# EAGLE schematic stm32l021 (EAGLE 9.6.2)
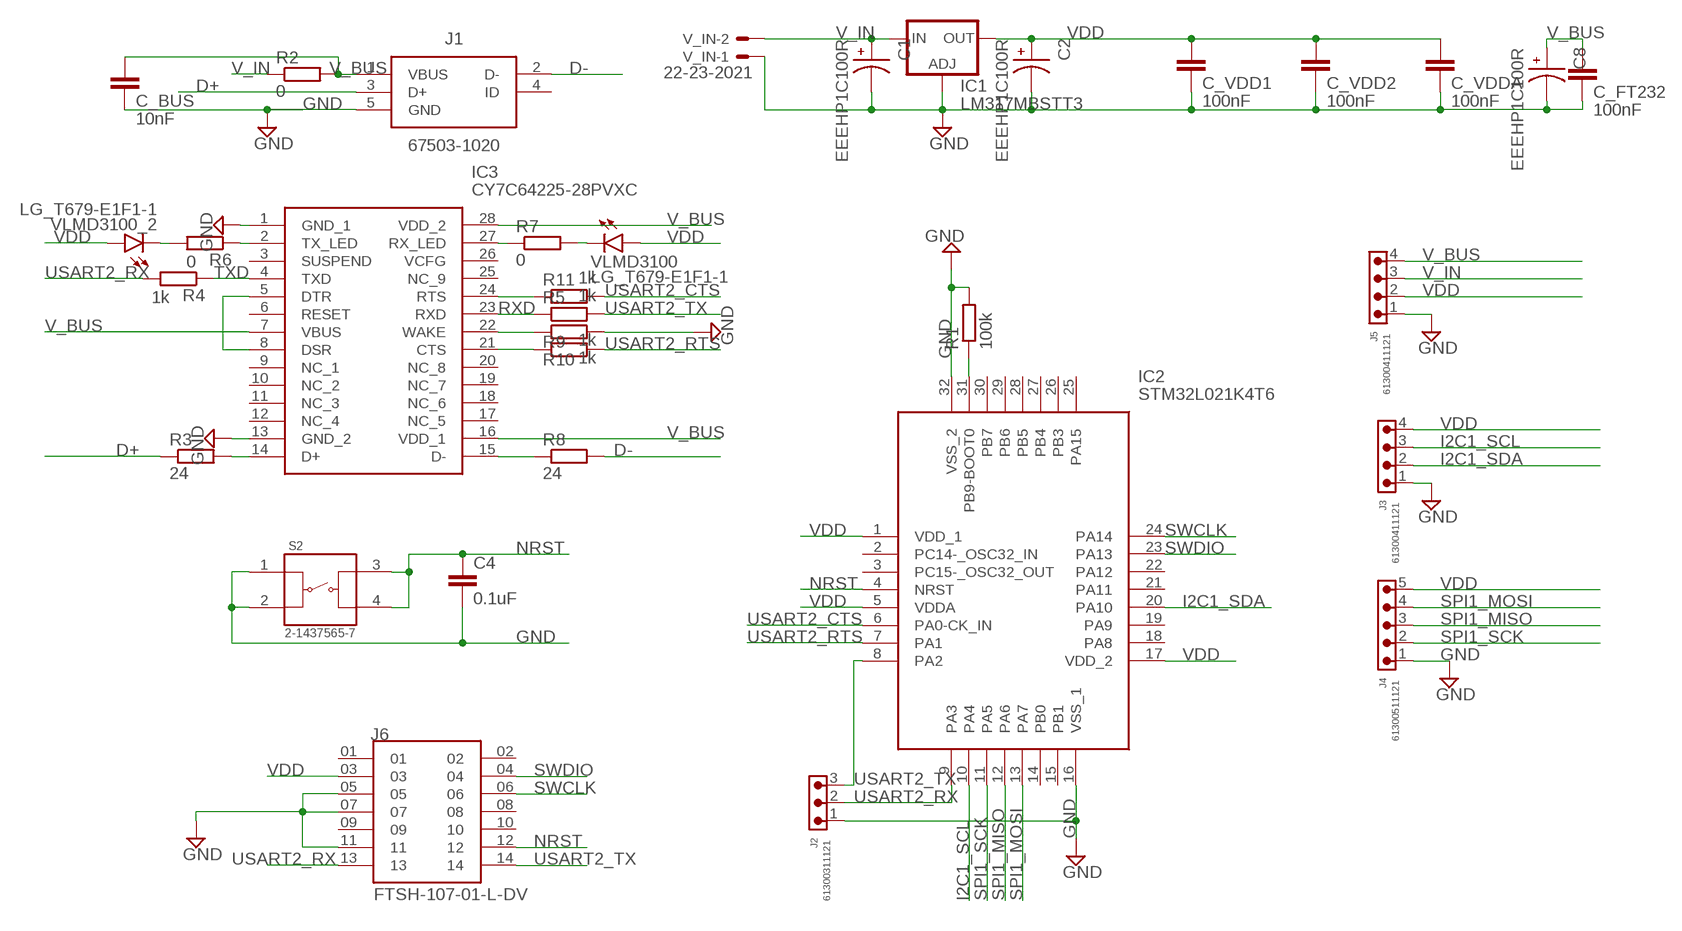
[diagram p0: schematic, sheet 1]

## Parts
C1  EEEHP1C100R  [CAP_EEEHP1C100R]
C2  EEEHP1C100R  [CAP_EEEHP1C100R]
C4  0.1uF  C-EUC0603  [C0603]
C8  EEEHP1C100R  [CAP_EEEHP1C100R]
C_BUS  10nF  C-EUC0603  [C0603]
C_FT232  100nF  C-EUC0603  [C0603]
C_VDD1  100nF  C-EUC0603  [C0603]
C_VDD2  100nF  C-EUC0603  [C0603]
C_VDDA  100nF  C-EUC0603  [C0603]
IC1  LM317MBSTT3  [SOT223]
IC2  STM32L021K4T6  [QFP80P900X900X160-32N]
IC3  CY7C64225-28PVXC  [SOP65P780X185-28N]
J1  67503-1020  [67503-1020]
J2  61300311121  6130XX11121_61300311121  [61300311121]
J3  61300411121  6130XX11121_61300411121  [61300411121]
J4  61300511121  6130XX11121_61300511121  [61300511121]
J5  61300411121  6130XX11121_61300411121  [61300411121]
J6  FTSH-107-01-L-DV  [SAMTEC_FTSH-107-01-L-DV]
R1  100k  R-EU_R0603  [R0603]
R2  0  R-EU_R0603  [R0603]
R3  24  R-EU_R0603  [R0603]
R4  1k  R-EU_R0603  [R0603]
R5  1k  R-EU_R0603  [R0603]
R6  0  R-EU_R0603  [R0603]
R7  0  R-EU_R0603  [R0603]
R8  24  R-EU_R0603  [R0603]
R9  1k  R-EU_R0603  [R0603]
R10  1k  R-EU_R0603  [R0603]
R11  1k  R-EU_R0603  [R0603]
S2  2-1437565-7  [SW_2-1437565-7]
V_IN  22-23-2021  [22-23-2021]
VLMD3100  LG_T679-E1F1-1  [PLCC2]
VLMD3100_2  LG_T679-E1F1-1  [PLCC2]

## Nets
D+: J1.3(D+) R3.1
D-: J1.2(D-) R8.2
GND: C1.2 C2.2 C4.2 C8.2 C_BUS.2 C_FT232.2 C_VDD1.2 C_VDD2.2 C_VDDA.2 IC1.1(ADJ) IC2.16(VSS_1) IC2.32(VSS_2) IC3.1(GND_1) IC3.13(GND_2) J1.5(GND) J2.1 J3.1 J4.1 J5.1 J6.05 J6.07 J6.11 R1.2 R9.2 S2.1 S2.2 V_IN.1
I2C1_SCL: IC2.10(PA4) J3.3
I2C1_SDA: IC2.20(PA10) J3.2
N$1: R6.2 VLMD3100_2.C
N$2: IC2.31(PB9-BOOT0) R1.1
N$3: IC3.2(TX_LED) R6.1
N$4: IC3.27(RX_LED) R7.1
N$5: IC3.14(D+) R3.2
N$6: R7.2 VLMD3100.C
N$7: IC3.5(DTR) IC3.8(DSR)
N$8: IC3.15(D-) R8.1
N$9: IC3.22(WAKE) R9.1
N$10: IC3.24(RTS) R11.1
N$11: IC3.21(CTS) R10.1
NRST: C4.1 IC2.4(NRST) J6.12 S2.3 S2.4
RXD: IC3.23(RXD) R5.1
SPI1_MISO: IC2.12(PA6) J4.3
SPI1_MOSI: IC2.13(PA7) J4.4
SPI1_SCK: IC2.11(PA5) J4.2
SWCLK: IC2.24(PA14) J6.06
SWDIO: IC2.23(PA13) J6.04
TXD: IC3.4(TXD) R4.1
USART2_CTS: IC2.6(PA0-CK_IN) R11.2
USART2_RTS: IC2.7(PA1) R10.2
USART2_RX: IC2.9(PA3) J2.2 J6.13 R4.2
USART2_TX: IC2.8(PA2) J2.3 J6.14 R5.2
V_BUS: C8.1 C_BUS.1 C_FT232.1 IC3.7(VBUS) IC3.16(VDD_1) IC3.28(VDD_2) J1.1(VBUS) J5.4 R2.2
V_IN: C1.1 IC1.3(IN) J5.3 R2.1 V_IN.2
VDD: C2.1 C_VDD1.1 C_VDD2.1 C_VDDA.1 IC1.4(OUT) IC2.1(VDD_1) IC2.5(VDDA) IC2.17(VDD_2) J3.4 J4.5 J5.2 J6.03 VLMD3100.A VLMD3100_2.A
Unconnected: IC2.2(PC14-_OSC32_IN) IC2.3(PC15-_OSC32_OUT) IC2.14(PB0) IC2.15(PB1) IC2.18(PA8) IC2.19(PA9) IC2.21(PA11) IC2.22(PA12) IC2.25(PA15) IC2.26(PB3) IC2.27(PB4) IC2.28(PB5) IC2.29(PB6) IC2.30(PB7) IC3.3(SUSPEND) IC3.6(RESET) IC3.9(NC_1) IC3.10(NC_2) IC3.11(NC_3) IC3.12(NC_4) IC3.17(NC_5) IC3.18(NC_6) IC3.19(NC_7) IC3.20(NC_8) IC3.25(NC_9) IC3.26(VCFG) J1.4(ID) J6.01 J6.02 J6.08 J6.09 J6.10

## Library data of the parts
C1 C2 C8 = EEEHP1C100R:EEEHP1C100R: Check availability; AVAILABILITY: In Stock; DESCRIPTION: Cap Aluminum Lytic 10uF 16V 20% (5 X 5.8mm) SMD 25mA 2000h 105C Automotive T/R; MF: Panasonic; MP: EEEHP1C100R; PACKAGE: RADIAL-2 Panasonic; PRICE: None; PURCHASE-URL: https://pricing.snapeda.com/search/part/EEEHP1C100R/?ref=eda
C4 C_BUS C_FT232 C_VDD1 C_VDD2 C_VDDA = rcl:C-EU: CAPACITOR, European symbol; SPICEPREFIX: C
IC1 = v-reg:LM317?*: 500 mA Adjustable Output Positive Voltage Regulator Source: http://www.onsemi.co.jp .. LM317M-D.PDF
IC2 = SamacSys_Parts:STM32L021K4T6: ARM Microcontrollers - MCU 16/32-BITS MICROS Source: Datasheet; DESCRIPTION: ARM Microcontrollers - MCU 16/32-BITS MICROS; HEIGHT: 1.6mm; MANUFACTURER_NAME: STMicroelectronics; MANUFACTURER_PART_NUMBER: STM32L021K4T6; MOUSER_PART_NUMBER: 511-STM32L021K4T6; MOUSER_PRICE-STOCK: https://www.mouser.co.uk/ProductDetail/STMicroelectronics/STM32L021K4T6?qs=dTJS0cRn7ohCWAWNqbLYkA%3D%3D
IC3 = CY7C64225-28PVXC:CY7C64225-28PVXC: Cypress Semiconductor CY7C64225-28PVXC, USB Controller, 12Mbit/s, USB 2.0, 3.3 V, 5 V, 28-Pin SSOP Source: Datasheet; DESCRIPTION: Cypress Semiconductor CY7C64225-28PVXC, USB Controller, 12Mbit/s, USB 2.0, 3.3 V, 5 V, 28-Pin SSOP; HEIGHT: 1.85mm; MANUFACTURER_NAME: Cypress Semiconductor; MANUFACTURER_PART_NUMBER: CY7C64225-28PVXC; MOUSER_PART_NUMBER: 727-CY7C64225-28PVXC; MOUSER_PRICE-STOCK: https://www.mouser.co.uk/ProductDetail/Cypress-Semiconductor/CY7C64225-28PVXC?qs=YrQxKq3BqGD638xSzFasMw%3D%3D
J1 = 67503-1020:67503-1020: 0.8mm USB OTG Mini B SMT R/A Sol Tab Molex On-The-Go Series Right Angle SMT Version 2.0 Type B Mini USB Connector, Receptacle, 30 V ac/dc, 1A Source: Datasheet Check availability; AVAILABILITY: In Stock; DESCRIPTION: USB - mini B USB 2.0 OTG Receptacle Connector 5 Position Surface Mount, Right Angle; MF: Molex; MP: 67503-1020; PACKAGE: None; PRICE: None; PURCHASE-URL: https://pricing.snapeda.com/search/part/67503-1020/?ref=eda
J2 = Eagle_WR-PHD (rev21a):6130XX11121_61300311121: WR-PHD 2.54 mm THT Pin Header ARTICLE PROPERTIES: Pins:1;​ 2;​ 3;​ 4;​ 5;​ 6;​ 7;​ 8;​ 9;​ 10;​ 12;​ 13;​ 14;​ 15;​ 16;​ 18;​ 20;​ 22;​ 24;​ 25;​ 32;​ 36;​ 40 KIND PROPERTIES: Pitch：2.54 mm Quality Class:3 as per CECC 75 301-802 Rows：Single Gender：Pin Header Type：Straight MATERIAL PROPERTIES: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; DATASHEET-URL: https://www.we-online.com/catalog/datasheet/61300311121.pdf; GENDER: Pin Header; IR: 3A; MOUNT: THT; PACKAGING: Bag; PART-NUMBER: 61300311121; PINS: 3; PITCH: 2.54mm; ROWS: Single; TYPE: Straight
J3 J5 = Eagle_WR-PHD (rev21a):6130XX11121_61300411121: WR-PHD 2.54 mm THT Pin Header ARTICLE PROPERTIES: Pins:1;​ 2;​ 3;​ 4;​ 5;​ 6;​ 7;​ 8;​ 9;​ 10;​ 12;​ 13;​ 14;​ 15;​ 16;​ 18;​ 20;​ 22;​ 24;​ 25;​ 32;​ 36;​ 40 KIND PROPERTIES: Pitch：2.54 mm Quality Class:3 as per CECC 75 301-802 Rows：Single Gender：Pin Header Type：Straight MATERIAL PROPERTIES: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; DATASHEET-URL: https://www.we-online.com/catalog/datasheet/61300411121.pdf; GENDER: Pin Header; IR: 3A; MOUNT: THT; PACKAGING: Bag; PART-NUMBER: 61300411121; PINS: 4; PITCH: 2.54mm; ROWS: Single; TYPE: Straight
J4 = Eagle_WR-PHD (rev21a):6130XX11121_61300511121: WR-PHD 2.54 mm THT Pin Header ARTICLE PROPERTIES: Pins:1;​ 2;​ 3;​ 4;​ 5;​ 6;​ 7;​ 8;​ 9;​ 10;​ 12;​ 13;​ 14;​ 15;​ 16;​ 18;​ 20;​ 22;​ 24;​ 25;​ 32;​ 36;​ 40 KIND PROPERTIES: Pitch：2.54 mm Quality Class:3 as per CECC 75 301-802 Rows：Single Gender：Pin Header Type：Straight MATERIAL PROPERTIES: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; DATASHEET-URL: https://www.we-online.com/catalog/datasheet/61300511121.pdf; GENDER: Pin Header; IR: 3A; MOUNT: THT; PACKAGING: Bag; PART-NUMBER: 61300511121; PINS: 5; PITCH: 2.54mm; ROWS: Single; TYPE: Straight
J6 = FTSH-107-01-L-DV:FTSH-107-01-L-DV; MANUFACTURER: Samtec; PARTREV: R; STANDARD: Manufacturer Recommendations
R1-R11 = rcl:R-EU_: RESISTOR, European symbol; SPICEPREFIX: R
S2 = 2-1437565-7:2-1437565-7: FSM2JSMA=SMT,TACTILE,PB SWITCH Check availability; AVAILABILITY: In Stock; COMMENT: 2-1437565-7; CONFIGURATION_POLE-THROW: Single Pole - Single Throw; CONTACT_CURRENT_RATING: 50 mA; DESCRIPTION: Tactile Switch SPST-NO Top Actuated Surface Mount; MF: TE Connectivity; MP: FSM2JSMA; PACKAGE: None; PRICE: None; PURCHASE-URL: https://pricing.snapeda.com/search/part/FSM2JSMA/?ref=eda
V_IN = con-molex:22-23-2021: .100" (2.54mm) Center Header - 2 Pin; MF: MOLEX; MPN: 22-23-2021; OC_FARNELL: 1462926; OC_NEWARK: 25C3832
VLMD3100 VLMD3100_2 = led:*_T679-?-1: LC TOPLED® Low Current LED; COLOR: green

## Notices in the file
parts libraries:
Eagle_WR-PHD: Copyright: Würth Elektronik
